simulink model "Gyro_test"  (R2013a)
settings: Solver=ode1  StartTime=0.0  StopTime=Inf  FixedStep=0.001  RelTol=1e-3
PostLoadFcn:
  | , if any(exist('dsrtsu_mdlpostloadfcn', 'file') == [2, 3, 6]), try dsrtsu_mdlpostloadfcn('Execute', bdroot); catch fprintf('Error in PostLoadFcn (dsrtsu_mdlpostloadfcn) for model "%s":\n %s\n', bdroot, lasterr); end, end,
libraries: rtilib1104 x1

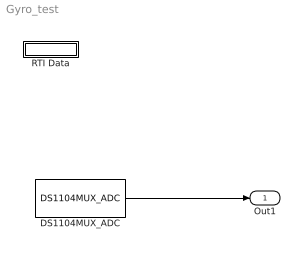
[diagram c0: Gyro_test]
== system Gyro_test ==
  DS1104MUX_ADC : rtilib1104/DS1104 MASTER PPC/DS1104MUX_ADC  ChannelNos=4  TriggerMode=0  Reserved1=[]  Reserved2=[]  Reserved3=[]  Reserved4=[]  DialogFcn=gui1104mux_adc  UnitName={ 'DS1104MUX_ADC' }  UnitValues={ [] }  DSProperties=struct('RTI',struct('Version',uint32(1),'BlockType',struct('isSLSource',uint8(1),'isSLSink',uint8(0),'isHWSource',uint8(1),'isHWSink',uint8(0),'isSetup',uint8(0),'isInline',uint8(1),'isNonInline',uint8(0),'isInterrupt',uint8(0),'isChannelwise',uint8(0)),'IOBoardType','DS1104MASTER','UnitType','ADC','Identifier','ADCMUX','DialogType','ML','BlockSet','NONE','SlaveProcessor','NONE'))
  RTI Data : Subsystem  Tag=struct('RTIDataServer',struct('RTIDataServerVs','2','RTIModelDescription','struct(''main'',''Gyro_test'',''sub'','''',''isMp'',0)'))  LoadFcn="if exist('rtidc'), try,  rtidc('DataHostBlockClbLoad', gcbh); catch, disp(['Warning: ''LoadFcn'' for RTI Data block failed: ' lasterr]); end, end,"
  Out1 : Outport
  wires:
  DS1104MUX_ADC/1 -> Out1/1

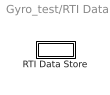
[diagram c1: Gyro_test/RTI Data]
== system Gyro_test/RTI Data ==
  RTI Data Store : Subsystem  Tag=struct('private',struct('version',struct('dsVer',uint32(2),'dsVerCreation',uint32(2),'RTI',struct('ver','7.0','type','RTI1104')),'access',struct('type','Model','isPerm',1,'created',['09-May-2014 14:17:55'],'modified',['09-May-2014 14:42:59'],'location','')),'public',struct('main',struct('data',[]),'sub',struct('name',{{'Gyro_test'}},'data',{{struct('TH',struct('thTaskInfo',struct('taskType',{'TIME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

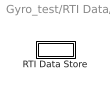
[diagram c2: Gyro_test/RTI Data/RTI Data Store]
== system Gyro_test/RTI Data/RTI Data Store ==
  RTI Data Store : Subsystem

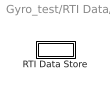
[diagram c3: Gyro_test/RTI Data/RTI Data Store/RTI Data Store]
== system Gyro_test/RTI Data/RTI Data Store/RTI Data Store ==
  RTI Data Store : Subsystem

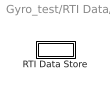
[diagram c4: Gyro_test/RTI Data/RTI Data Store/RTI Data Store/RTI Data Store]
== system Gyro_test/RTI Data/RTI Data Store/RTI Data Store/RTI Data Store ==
  RTI Data Store : Subsystem

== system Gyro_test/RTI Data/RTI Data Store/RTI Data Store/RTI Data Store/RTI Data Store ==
